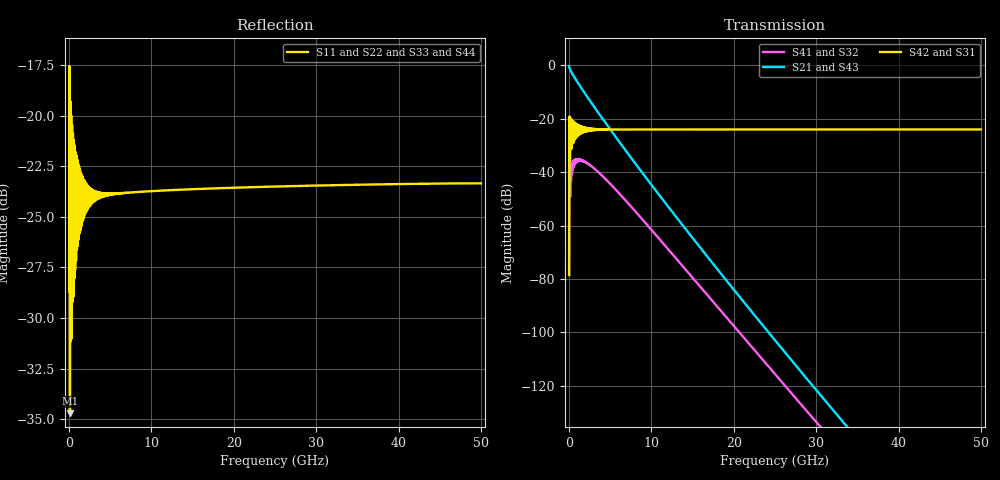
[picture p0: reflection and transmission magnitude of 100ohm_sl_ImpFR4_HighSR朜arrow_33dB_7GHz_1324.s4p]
# GHz S RI R 50
! S-Parameters data
! Freq  reS11  imS11  reS12  imS12  reS13  imS13  reS14  imS14
!  reS21  imS21  reS22  imS22  reS23  imS23  reS24  imS24
!  reS31  imS31  reS32  imS32  reS33  imS33  reS34  imS34
!  reS41  imS41  reS42  imS42  reS43  imS43  reS44  imS44
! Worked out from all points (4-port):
!   5001 points, 1 Hz to 50 GHz, reference 50 ohm
!   strongest paths, dB at 1 Hz, 12.5 GHz, 25 GHz, 37.5 GHz, 50 GHz:
!     S42: -78.5, -24.0, -24.0, -24.0, -24.0
!     S31: -78.5, -24.0, -24.0, -24.0, -24.0
!     S21: -0.3, -54.8, -103.0, -149.1, -193.0
!     S43: -0.3, -54.8, -103.0, -149.1, -193.0
!     S41: -78.5, -70.6, -115.7, -160.1, -
!     S32: -78.5, -70.6, -115.7, -160.1, -
!   lowest |S11| = -34.7 dB at 100 MHz (marker M1), VSWR 1.04, Z = 51.7 - j0.802 ohm
!   |S11| at or under -10 dB: start of sweep to end of sweep
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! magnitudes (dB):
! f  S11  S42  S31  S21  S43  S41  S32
! 1 Hz  -28.7  -78.5  -78.5  -0.3  -0.3  -78.5  -78.5
! 100 MHz  -34.7  -35.8  -35.8  -1.4  -1.4  -40.7  -40.7
! 260 MHz  -20.0  -20.2  -20.2  -2.5  -2.5  -39.3  -39.3
! 1.79 GHz  -24.9  -24.9  -24.9  -9.9  -9.9  -35.8  -35.8
! 15.01 GHz  -23.6  -24.0  -24.0  -64.7  -64.7  -79.6  -79.6
! 19 GHz  -23.6  -24.0  -24.0  -80.2  -80.2  -94.0  -94.0
! 50 GHz  -23.3  -24.0  -24.0  -193.0  -193.0  -  -
